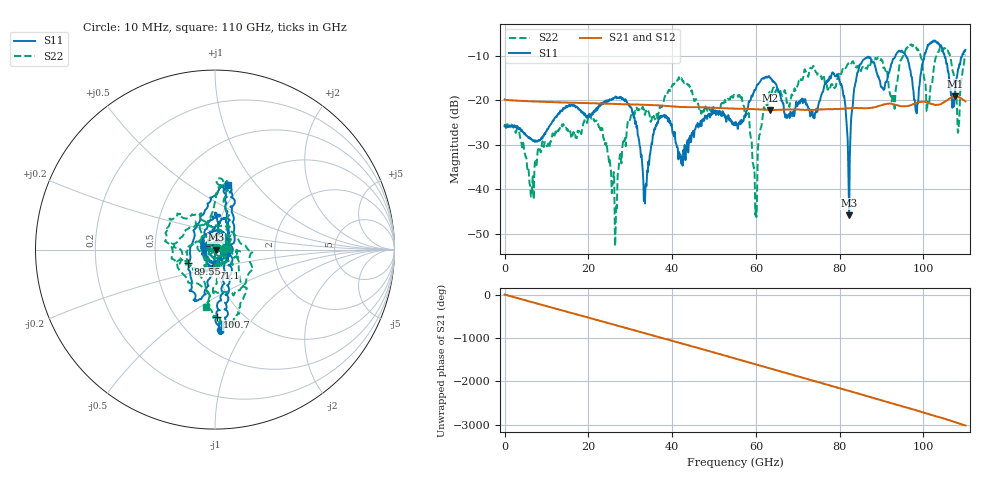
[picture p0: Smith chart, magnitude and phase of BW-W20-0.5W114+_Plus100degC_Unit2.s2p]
!Mini-Circuits Laboratory
!S-Parameters
!Model: BW-W20-0.5W114+
!Run / Lot / Date Code: QN2409253 /  / N/A
!Fixture:
!Network Analyzer: PNA-X N5242B - 423 4 ports (COM/DCOM);  Serial number: 74408
!Date: 3/8/2024 at 1:33:03 PM
!No.: Unit# 6 (U2  100C)
!Tested with:
# Hz  S  dB  R  50
!Frequency  S11 dB  S11 Deg  S21 dB  S21 Deg  S12 dB  S12 Deg  S22 dB  S22 Deg
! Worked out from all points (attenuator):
!   2208 points, 10 MHz to 110 GHz, reference 50 ohm
!   highest |S21| = -19.14 dB at 107.6 GHz (marker M1); lowest = -22.2 dB at 63.35 GHz (marker M2)
!   lowest |S11| = -45.9 dB at 82.25 GHz (marker M3), VSWR 1.01, Z = 50.5 - j0.081 ohm
!   |S11| at or under -10 dB: start of sweep to 93.3 GHz; 95.81 GHz to 100.2 GHz (4.397 GHz wide, 4.49 % of centre); 105 GHz to 109.2 GHz (4.193 GHz wide, 3.91 % of centre)
!   |S22| runs from -52.8 to -7.4 dB; largest |S21 - S12| = 0.0027
!   S11 on the Smith chart (normalised r, x): 10 MHz: 1.11, +0.00; 71.1 GHz: 0.95, -0.19; 89.55 GHz: 0.73, -0.12; 100.7 GHz: 0.77, -0.67; 110 GHz: 0.87, +0.73
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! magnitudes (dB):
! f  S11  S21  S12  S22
! 10 MHz  -25.8  -19.8  -19.8  -25.7
! 6.45 GHz  -28.8  -20.2  -20.2  -41.4
! 18.35 GHz  -22.7  -20.6  -20.6  -27.5
! 22.9 GHz  -21.1  -20.7  -20.7  -27.0
! 26.35 GHz  -19.3  -20.8  -20.8  -52.8
! 33.5 GHz  -43.2  -21.0  -21.0  -23.3
! 36.7 GHz  -24.5  -21.1  -21.2  -23.2
! 55.05 GHz  -25.6  -21.9  -21.9  -18.8
! 59.8 GHz  -17.8  -22.0  -22.0  -43.4
! 63.35 GHz  -15.0  -22.2  -22.2  -18.4
! 71.1 GHz  -19.9  -22.1  -22.2  -15.4
! 73.35 GHz  -22.7  -22.2  -22.2  -12.8
! 79.3 GHz  -14.3  -22.0  -21.9  -15.5
! 82.25 GHz  -45.9  -21.8  -21.7  -11.6
! 84.95 GHz  -11.8  -21.7  -21.8  -13.3
! 89.55 GHz  -15.5  -21.2  -21.4  -10.8
! 91.7 GHz  -13.9  -20.7  -20.8  -17.0
! 98.25 GHz  -22.4  -20.6  -20.7  -8.1
! 100.7 GHz  -8.5  -20.5  -20.4  -21.6
! 104.4 GHz  -8.3  -20.7  -20.7  -8.8
! 107.6 GHz  -17.1  -19.1  -19.2  -18.3
! 110 GHz  -8.6  -20.2  -20.3  -9.7
